(* Logix 5000 AddOnInstructionDefinition export AMCI_SMD34E2_Run_Dwell_Move; software revision 20.03 *)

ADD_ON_INSTRUCTION AMCI_SMD34E2_Run_Dwell_Move   (* revision 1.0, vendor AMCI *)
VAR_INPUT
   Type_0_for_standard_1_for_indexed : BOOL;
   Assembled_Move_Dwell_Timer : INT; {required}
END_VAR
VAR_IN_OUT
   AMCI_SMD34E2_output_data : _000A:SMD34E2_788832CB:O:0; {required}
END_VAR
VAR
   command_data_block : INT[10];
        [0]   // Command Bits MSW
        [1]   // Command Bits LSW
        [2]   // Upper Target Position
        [3]   // Lower Target Position
        [4]   // Upper Programmed Speed
        [5]   // Lower Programmed Speed
END_VAR

ROUTINE Logic   (* ladder *)
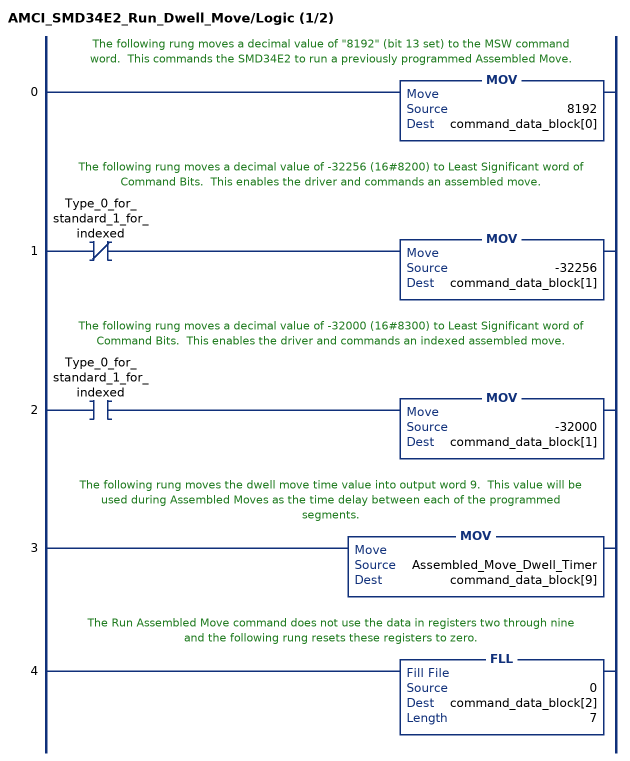
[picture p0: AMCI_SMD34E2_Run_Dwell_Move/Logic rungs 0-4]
   // The following rung moves a decimal value of "8192" (bit 13 set) to the MSW command word.  This commands the SMD34E2 to run a previously programmed Assembled Move.
   0: MOV(8192,command_data_block[0]);
   // The following rung moves a decimal value of -32256 (16#8200) to Least Significant word of Command Bits.  This enables the driver and commands an assembled move.
   1: XIO(Type_0_for_standard_1_for_indexed)MOV(-32256,command_data_block[1]);
   // The following rung moves a decimal value of -32000 (16#8300) to Least Significant word of Command Bits.  This enables the driver and commands an indexed assembled move.
   2: XIC(Type_0_for_standard_1_for_indexed)MOV(-32000,command_data_block[1]);
   // The following rung moves the dwell move time value into output word 9.  This value will be used during Assembled Moves as the time delay between each of the programmed segments.
   3: MOV(Assembled_Move_Dwell_Timer,command_data_block[9]);
   // The Run Assembled Move command does not use the data in registers two through nine and the following rung resets these registers to zero.
   4: FLL(0,command_data_block[2],7);
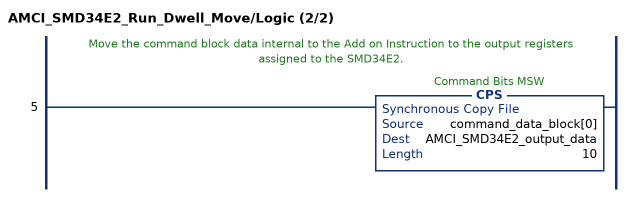
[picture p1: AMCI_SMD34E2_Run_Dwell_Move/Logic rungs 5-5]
   // Move the command block data internal to the Add on Instruction to the output registers assigned to the SMD34E2.
   5: CPS(command_data_block[0],AMCI_SMD34E2_output_data,10);
END_ROUTINE
END_ADD_ON_INSTRUCTION
